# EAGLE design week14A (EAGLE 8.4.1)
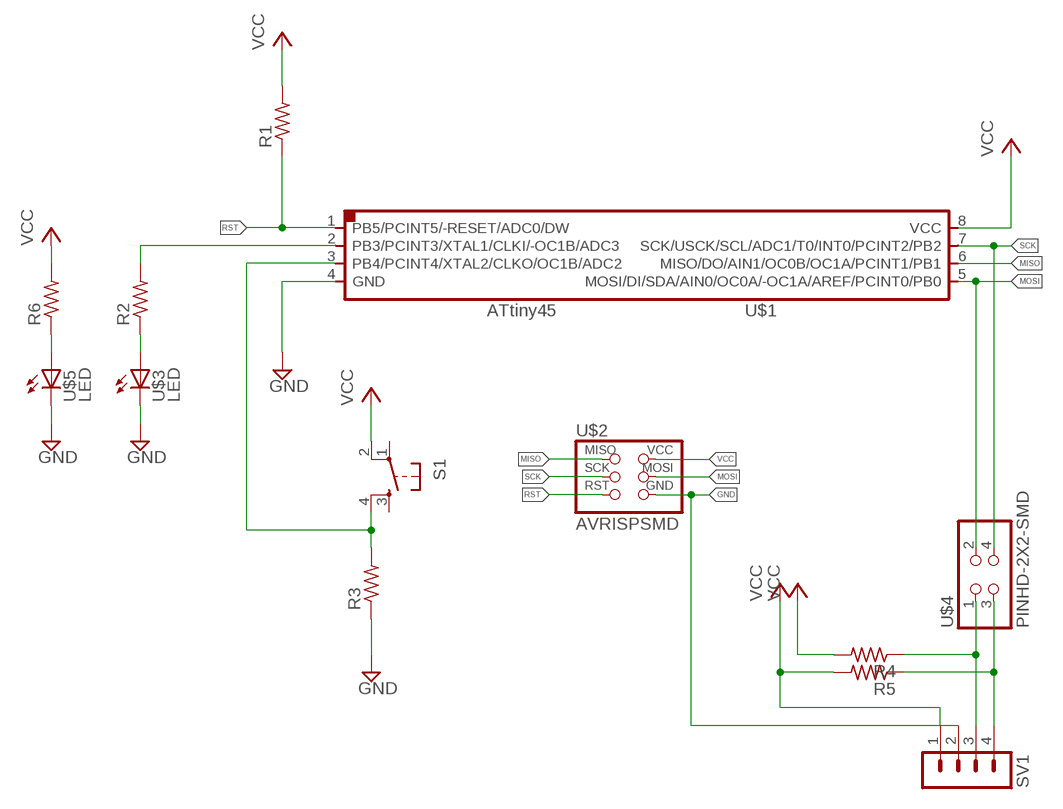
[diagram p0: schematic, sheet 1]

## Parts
R1  RES-US1206  [R1206]
R2  RES-US1206  [R1206]
R3  RES-US1206  [R1206]
R4  RES-US1206  [R1206]
R5  RES-US1206  [R1206]
R6  RES-US1206  [R1206]
S1  6MM_SWITCH6MM_SWITCH  [6MM_SWITCH]
SV1  MA04-1  [MA04-1]
U$1  ATTINY45SI  [SOIC8]
U$2  AVRISPSMD  [2X03SMD]
U$3  LED  [LED1206]
U$4  PINHD-2X2-SMD  [2X02SMD]
U$5  LED  [LED1206]

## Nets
GND: R3.1 SV1.2 U$1.4(GND) U$2.6(GND) U$3.2(C) U$5.2(C)
MISO: U$1.6(MISO/DO/AIN1/OC0B/OC1A/PCINT1/PB1) U$2.1(MISO)
MOSI: U$1.5(MOSI/DI/SDA/AIN0/OC0A/-OC1A/AREF/PCINT0/PB0) U$2.4(MOSI) U$4.2
N$1: R2.2 U$1.2(PB3/PCINT3/XTAL1/CLKI/-OC1B/ADC3)
N$3: R2.1 U$3.1(A)
N$4: R3.2 S1.4(S1) U$1.3(PB4/PCINT4/XTAL2/CLKO/OC1B/ADC2)
N$5: R4.1 SV1.3 U$4.1
N$6: R5.1 SV1.4 U$4.3
N$7: R6.1 U$5.1(A)
RST: R1.1 U$1.1(PB5/PCINT5/-RESET/ADC0/DW) U$2.5(RST)
SCK: U$1.7(SCK/USCK/SCL/ADC1/T0/INT0/PCINT2/PB2) U$2.3(SCK) U$4.4
VCC: R1.2 R4.2 R5.2 R6.2 S1.2(P1) SV1.1 U$1.8(VCC) U$2.2(VCC)
Unconnected: S1.1(P) S1.3(S)

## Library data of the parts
R1-R6 = fab:RES-US: Resistor (US Symbol)
S1 = fab:6MM_SWITCH: OMRON SWITCH
SV1 = con-lstb:MA04-1: PIN HEADER; OC_FARNELL: unknown; OC_NEWARK: unknown
U$1 = fab:ATTINY45
U$2 = fab:AVRISP
U$3 U$5 = fab:LED: LED
U$4 = fab:PINHD-2X2-SMD

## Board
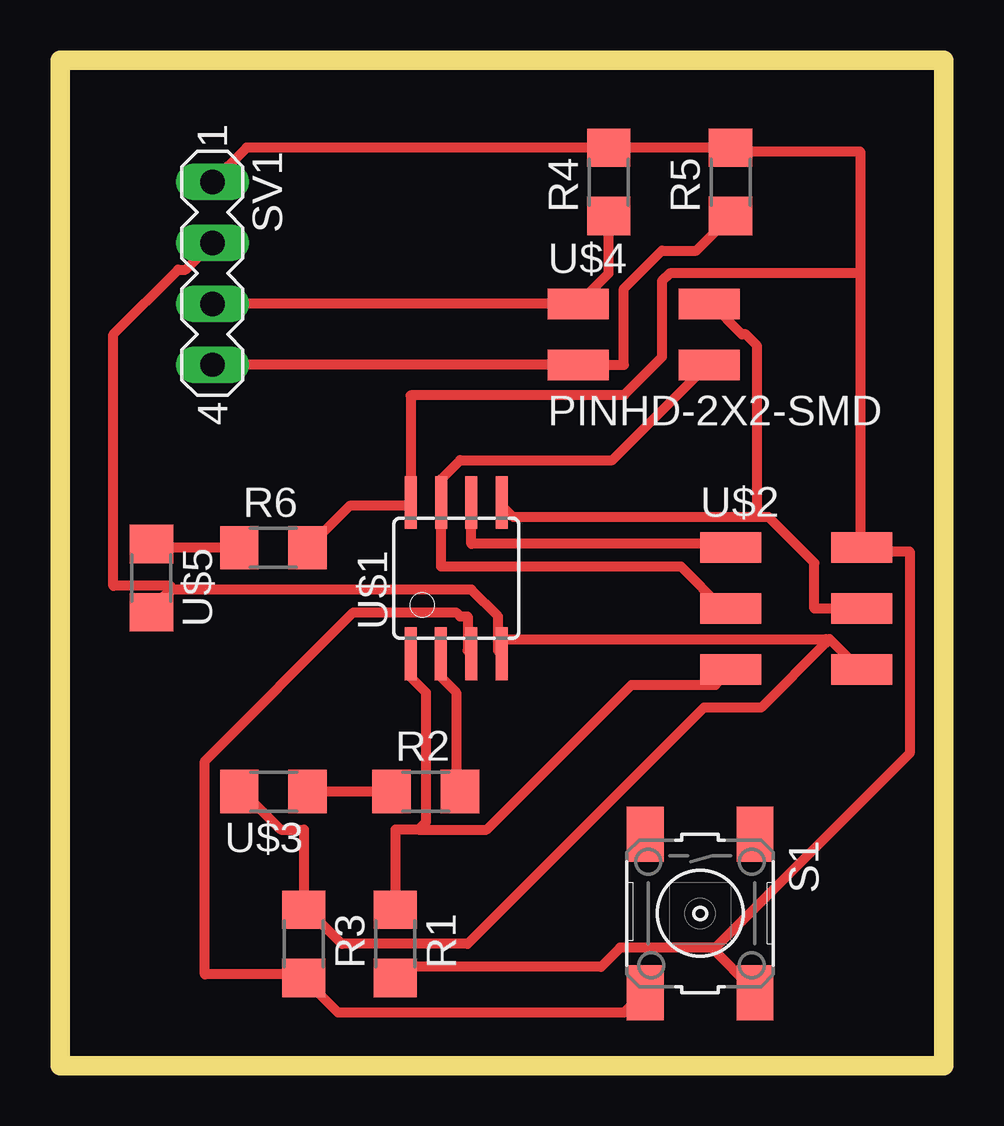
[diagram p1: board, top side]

Size 36.83 x 41.91 mm. Coordinates in mm from the lower left corner, seen from the top.
Outline: 0,0 36.81,0 36.81,41.58 0,41.58 0,0
Outline: 0,0 36.83,0 36.83,41.91 0,41.91 0,0
Copper layers (1*16): Top 0.035mm / dielectric 1.5mm / Bottom 0.035mm
Design rules "default *": minimum track width 16mil, minimum drill 0.35mm, track to track 16mil, track to pad 16mil, pad to pad 16mil, via to via 6mil, smd to smd 16mil, copper to edge 16mil, drill to drill 16mil, minimum pad ring 10mil, minimum via ring 8mil, stop-mask expansion 4mil, vias tented up to drill 0mil, thermal gap 10mil

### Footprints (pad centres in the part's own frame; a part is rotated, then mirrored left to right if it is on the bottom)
R1206 = smd 1.6 x 1.803: 1 -1.422,0; 2 1.422,0
6MM_SWITCH = smd 2.286 x 1.524: 1 -3.302,2.286; 2 3.302,2.286; 3 -3.302,-2.286; 4 3.302,-2.286
MA04-1 = drill 1.016 long: 1 -3.81,0; 2 -1.27,0; 3 1.27,0; 4 3.81,0
SOIC8 = smd 0.5 x 2.2: 1 -1.905,-3.154; 2 -0.645,-3.154; 3 0.625,-3.154; 4 1.895,-3.154; 5 1.905,3.154; 6 0.635,3.154; 7 -0.635,3.154; 8 -1.905,3.154
2X03SMD = smd 2.54 x 1.27: 1 -2.54,2.54; 2 2.92,2.54; 3 -2.54,0; 4 2.92,0; 5 -2.54,-2.54; 6 2.92,-2.54
LED1206 = smd 1.6 x 1.803: 1 -1.422,0; 2 1.422,0
2X02SMD = smd 2.54 x 1.27: 1 -2.54,1.27; 2 2.92,1.27; 3 -2.54,-1.27; 4 2.92,-1.27

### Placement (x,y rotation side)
R1  13.97,5.08 270 top
R2  15.24,11.43 0 top
R3  10.16,5.08 270 top
R4  22.86,36.83 90 top
R5  27.94,36.83 90 top
R6  8.89,21.59 0 top
S1  26.67,6.35 270 top
SV1  6.35,33.02 270 top
U$1  16.51,20.32 0 top
U$2  30.48,19.05 0 top
U$3  8.89,11.43 180 top
U$4  24.13,30.48 0 top
U$5  3.81,20.32 270 top

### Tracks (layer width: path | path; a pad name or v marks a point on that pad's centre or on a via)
GND
  Top 0.406: U$3.2 7.62,11.43 9.21,9.84 10.16,9.84 R3.1 10.32,6.51 11.75,5.08 16.99,5.08 26.83,14.92 29.21,14.92 31.91,17.62 31.91,17.78 | 4.6,19.84 3.81,19.05 U$5.2 | 4.6,19.84 17.14,19.84 18.26,18.73 18.26,17.3 U$1.4 18.41,17.78 31.91,17.78 | 31.91,17.78 32.07,17.78 33.34,16.51 U$2.6 | SV1.2 5.24,33.18 4.92,33.18 2.22,30.48 2.22,20 4.6,20 4.6,19.84
MISO
  Top 0.406: U$1.6 17.14,21.75 27.78,21.75 U$2.1
MOSI
  Top 0.406: 29.05,22.86 29.53,22.86 31.43,20.96 31.43,19.05 U$2.4 | 29.05,22.86 18.89,22.86 18.41,23.34 U$1.5 | 29.05,22.86 29.05,30 28.57,30.48 28.42,30.48 27.15,31.75 U$4.2
N$1
  Top 0.406: R2.2 16.51,11.43 16.51,15.56 15.88,16.19 15.88,17.14 U$1.2
N$3
  Top 0.406: R2.1 U$3.1
N$4
  Top 0.406: S1.4 24.29,3.02 23.49,2.22 11.59,2.22 R3.2 10.16,3.81 6.03,3.81 6.03,12.7 12.22,18.89 16.51,18.89 16.67,18.73 16.99,18.73 16.99,17.3 U$1.3
N$5
  Top 0.406: R4.1 22.86,33.02 U$4.1 SV1.3
N$6
  Top 0.406: R5.1 26.51,33.97 25.08,33.97 23.49,32.39 23.49,29.21 U$4.3 SV1.4
N$7
  Top 0.406: R6.1 3.81,21.59 U$5.1
RST
  Top 0.406: R1.1 13.97,9.84 14.92,9.84 | 14.92,9.84 15.24,10.16 15.24,15.56 14.6,16.19 U$1.1 | U$2.5 27.3,15.88 23.81,15.88 17.78,9.84 14.92,9.84
SCK
  Top 0.406: U$2.3 27.62,19.05 25.88,20.8 15.88,20.8 U$1.7 15.88,24.45 16.67,25.24 23.02,25.24 26.99,29.21 U$4.4
VCC
  Top 0.406: 27.15,4.92 23.34,4.92 22.54,4.13 14.29,4.13 13.97,3.81 R1.2 | 27.15,4.92 28.89,3.18 S1.2 | R6.2 12.06,23.34 14.6,23.34 U$1.8 14.6,27.94 23.49,27.94 25.08,29.53 25.08,32.7 25.4,33.02 33.34,33.02 | 33.34,33.02 33.34,38.1 27.94,38.1 R5.2 R4.2 22.7,38.26 7.78,38.26 SV1.1 | 33.34,33.02 33.34,21.59 U$2.2 33.5,21.43 35.4,21.43 35.4,13.02 27.3,4.92 27.15,4.92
